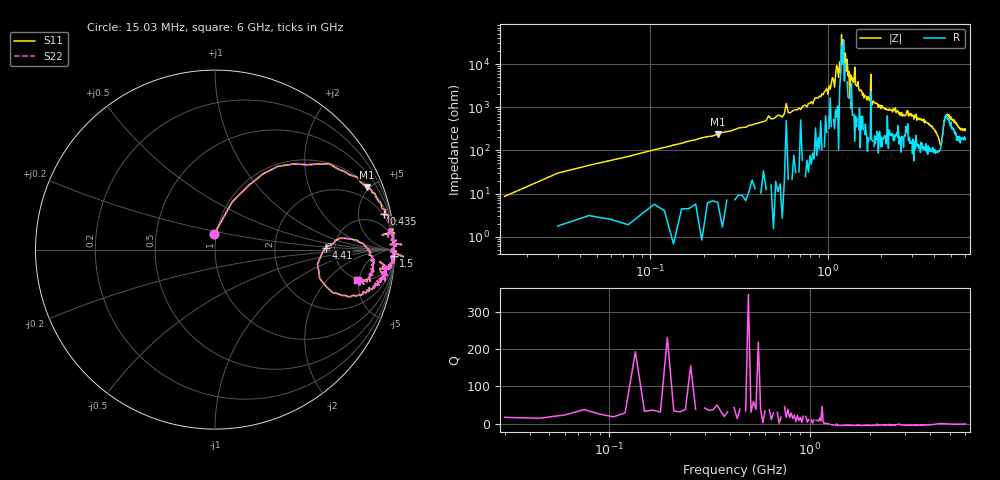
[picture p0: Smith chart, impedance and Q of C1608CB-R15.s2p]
!	Network	Analyzer	HP8753E.07.74:	Oct	30	2002	Serial	No.	JP38451487
!	Hewlett-Packard
!	7	Sep	2009	10:01:29
!	Frequency	S11	S21	S12	S22
#	HZ	S	RI	R	50
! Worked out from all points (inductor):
!   400 points, 15.03 MHz to 6 GHz, reference 50 ohm
!   read as one part in series: L = 156 nH near 45.03 MHz
!   highest Q = 38 at 240 MHz (marker M1), where L = 159 nH
!   self-resonance near 1.215 GHz
!   S11 on the Smith chart (normalised r, x): 15.03 MHz: 0.98, +0.17; 435 MHz: 1.66, +9.29; 1.5 GHz: 6, -54; 4.41 GHz: 4.22, +0.16; 6 GHz: 4.74, -4.74
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1.502992e7  -0.00412 0.0868  1 -0.0868  1 -0.0868  -0.00412 0.0868
6.00297e7  0.268 0.422  0.732 -0.422  0.732 -0.422  0.268 0.422
2.400288e8  0.845 0.349  0.155 -0.349  0.155 -0.349  0.845 0.349
4.350278e8  0.943 0.199  0.0573 -0.199  0.0573 -0.199  0.943 0.199
1.020025e9  0.996 0.0316  0.00433 -0.0316  0.00433 -0.0316  0.996 0.0316
1.185024e9  0.985 0.00504  0.0148 -0.00504  0.0148 -0.00504  0.985 0.00504
1.200024e9  0.999 0.00171  0.00116 -0.00171  0.00116 -0.00171  0.999 0.00171
1.230024e9  0.997 -0.000488  0.00269 0.000488  0.00269 0.000488  0.997 -0.000488
1.245024e9  0.981 -0.00977  0.0193 0.00977  0.0193 0.00977  0.981 -0.00977
1.290024e9  0.998 -0.00735  0.00235 0.00735  0.00235 0.00735  0.998 -0.00735
1.335023e9  1.05 -0.0397  -0.0508 0.0397  -0.0508 0.0397  1.05 -0.0397
1.425023e9  1 -0.0118  0.000367 0.0118  0.000367 0.0118  1 -0.0118
1.500022e9  0.995 -0.0363  0.00549 0.0363  0.00549 0.0363  0.995 -0.0363
1.740021e9  0.987 -0.0658  0.0128 0.0658  0.0128 0.0658  0.987 -0.0658
1.755021e9  0.993 -0.0157  0.00705 0.0157  0.00705 0.0157  0.993 -0.0157
1.785021e9  0.979 -0.0845  0.0206 0.0845  0.0206 0.0845  0.979 -0.0845
2.01002e9  0.975 -0.0876  0.0254 0.0876  0.0254 0.0876  0.975 -0.0876
3.015015e9  0.961 -0.141  0.0395 0.141  0.0395 0.141  0.961 -0.141
4.00501e9  0.842 -0.243  0.158 0.243  0.158 0.243  0.842 -0.243
4.410008e9  0.617 0.0116  0.383 -0.0116  0.383 -0.0116  0.617 0.0116
5.010005e9  0.876 -0.107  0.124 0.107  0.124 0.107  0.876 -0.107
6e9  0.793 -0.171  0.207 0.171  0.207 0.171  0.793 -0.171
